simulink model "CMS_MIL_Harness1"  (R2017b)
settings: Solver=FixedStepDiscrete  StartTime=0.0  StopTime=23  FixedStep=0.01  RelTol=1e-3  EnableMultiTasking=on
undefined symbols (not defined in the file): sigbuilder_block
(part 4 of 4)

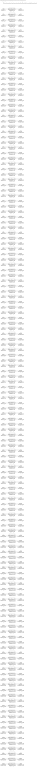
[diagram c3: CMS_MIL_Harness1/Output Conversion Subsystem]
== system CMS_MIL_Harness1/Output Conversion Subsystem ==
  note: This subsystem has been inserted by Simulink to adapt the output of the harnessed component to the interface required by the sink blocks. Modifying the contents of this subsystem may result in compilation and simulation failure.
  Inport_1 : Inport
  Inport_2 : Inport  Port=2
  Inport_3 : Inport  Port=3
  Inport_4 : Inport  Port=4
  Inport_5 : Inport  Port=5
  Inport_6 : Inport  Port=6
  Inport_7 : Inport  Port=7
  Inport_8 : Inport  Port=8
  Inport_9 : Inport  Port=9
  Inport_10 : Inport  Port=10
  Inport_11 : Inport  Port=11
  Inport_12 : Inport  Port=12
  Inport_13 : Inport  Port=13
  Inport_14 : Inport  Port=14
  Inport_15 : Inport  Port=15
  Inport_16 : Inport  Port=16
  Inport_17 : Inport  Port=17
  Inport_18 : Inport  Port=18
  Inport_19 : Inport  Port=19
  Inport_20 : Inport  Port=20
  Inport_21 : Inport  Port=21
  Inport_22 : Inport  Port=22
  Inport_23 : Inport  Port=23
  Inport_24 : Inport  Port=24
  Inport_25 : Inport  Port=25
  Inport_26 : Inport  Port=26
  Inport_27 : Inport  Port=27
  Inport_28 : Inport  Port=28
  Inport_29 : Inport  Port=29
  Inport_30 : Inport  Port=30
  Inport_31 : Inport  Port=31
  Inport_32 : Inport  Port=32
  Inport_33 : Inport  Port=33
  Inport_34 : Inport  Port=34
  Inport_35 : Inport  Port=35
  Inport_36 : Inport  Port=36
  Inport_37 : Inport  Port=37
  Inport_38 : Inport  Port=38
  Inport_39 : Inport  Port=39
  Inport_40 : Inport  Port=40
  Inport_41 : Inport  Port=41
  Inport_42 : Inport  Port=42
  Inport_43 : Inport  Port=43
  Inport_44 : Inport  Port=44
  Inport_45 : Inport  Port=45
  Inport_46 : Inport  Port=46
  Inport_47 : Inport  Port=47
  Inport_48 : Inport  Port=48
  Inport_49 : Inport  Port=49
  Inport_50 : Inport  Port=50
  Inport_51 : Inport  Port=51
  Inport_52 : Inport  Port=52
  Inport_53 : Inport  Port=53
  Inport_54 : Inport  Port=54
  Inport_55 : Inport  Port=55
  Inport_56 : Inport  Port=56
  Inport_57 : Inport  Port=57
  Inport_58 : Inport  Port=58
  Inport_59 : Inport  Port=59
  Inport_60 : Inport  Port=60
  Inport_61 : Inport  Port=61
  Inport_62 : Inport  Port=62
  Inport_63 : Inport  Port=63
  Inport_64 : Inport  Port=64
  Inport_65 : Inport  Port=65
  Inport_66 : Inport  Port=66
  Inport_67 : Inport  Port=67
  Inport_68 : Inport  Port=68
  Inport_69 : Inport  Port=69
  Inport_70 : Inport  Port=70
  Inport_71 : Inport  Port=71
  Inport_72 : Inport  Port=72
  Inport_73 : Inport  Port=73
  Inport_74 : Inport  Port=74
  Inport_75 : Inport  Port=75
  Inport_76 : Inport  Port=76
  Inport_77 : Inport  Port=77
  Inport_78 : Inport  Port=78
  Inport_79 : Inport  Port=79
  Inport_80 : Inport  Port=80
  Inport_81 : Inport  Port=81
  Inport_82 : Inport  Port=82
  Inport_83 : Inport  Port=83
  Inport_84 : Inport  Port=84
  Inport_85 : Inport  Port=85
  Inport_86 : Inport  Port=86
  Inport_87 : Inport  Port=87
  Inport_88 : Inport  Port=88
  Inport_89 : Inport  Port=89
  Inport_90 : Inport  Port=90
  Inport_91 : Inport  Port=91
  Inport_92 : Inport  Port=92
  Inport_93 : Inport  Port=93
  Inport_94 : Inport  Port=94
  Inport_95 : Inport  Port=95
  Inport_96 : Inport  Port=96
  Inport_97 : Inport  Port=97
  Inport_98 : Inport  Port=98
  Inport_99 : Inport  Port=99
  Inport_100 : Inport  Port=100
  Inport_101 : Inport  Port=101
  Inport_102 : Inport  Port=102
  Inport_103 : Inport  Port=103
  Inport_104 : Inport  Port=104
  Inport_105 : Inport  Port=105
  Inport_106 : Inport  Port=106
  Inport_107 : Inport  Port=107
  Inport_108 : Inport  Port=108
  Inport_109 : Inport  Port=109
  Inport_110 : Inport  Port=110
  Inport_111 : Inport  Port=111
  Inport_112 : Inport  Port=112
  Inport_113 : Inport  Port=113
  Inport_114 : Inport  Port=114
  Inport_115 : Inport  Port=115
  Inport_116 : Inport  Port=116
  Inport_117 : Inport  Port=117
  Inport_118 : Inport  Port=118
  Inport_119 : Inport  Port=119
  Inport_120 : Inport  Port=120
  Inport_121 : Inport  Port=121
  Inport_122 : Inport  Port=122
  Inport_123 : Inport  Port=123
  Inport_124 : Inport  Port=124
  Inport_125 : Inport  Port=125
  Inport_126 : Inport  Port=126
  Inport_127 : Inport  Port=127
  Inport_128 : Inport  Port=128
  Inport_129 : Inport  Port=129
  Inport_130 : Inport  Port=130
  Inport_131 : Inport  Port=131
  Inport_132 : Inport  Port=132
  Inport_133 : Inport  Port=133
  Inport_134 : Inport  Port=134
  Inport_135 : Inport  Port=135
  Inport_136 : Inport  Port=136
  Inport_137 : Inport  Port=137
  Inport_138 : Inport  Port=138
  Inport_139 : Inport  Port=139
  Inport_140 : Inport  Port=140
  Inport_141 : Inport  Port=141
  Inport_142 : Inport  Port=142
  Inport_143 : Inport  Port=143
  SigSpec_{1,6,16..17,22,36..38,41..42,46,57..59,66,78,85..87,135..136,138..140,142..143} (26 alike) : SignalSpecification  OutDataTypeStr=uint8  Unit=enum  Dimensions=[1]  SampleTime=0.01
  SigSpec_{2..5,8,10..11,29,34..35,40,49..52,55..56,67..77,79..83,90,92,97} (36 alike) : SignalSpecification  OutDataTypeStr=boolean  Unit=flg  Dimensions=[1]  SampleTime=0.01
  SigSpec_{100..114,119,127..134} (24 alike) : SignalSpecification  OutDataTypeStr=uint8  Unit=numb  Dimensions=[1]  SampleTime=0.01
  SigSpec_{25,28,115..118} (6 alike) : SignalSpecification  OutDataTypeStr=fixdt('ufix16_Sp001')  Unit=V  Dimensions=[1]  SampleTime=0.01
  SigSpec_{12..13,23..24,26..27,88,93..94,120..126} (16 alike) : SignalSpecification  OutDataTypeStr=fixdt('ufix8_Bn40')  Unit=C  Dimensions=[1]  SampleTime=0.01
  SigSpec_137 : SignalSpecification  OutDataTypeStr=boolean  Unit=flag  Dimensions=[1]  SampleTime=0.01
  SigSpec_14 : SignalSpecification  OutDataTypeStr=fixdt('ufix16_Sp1')  Unit=W  Dimensions=[1]  SampleTime=0.01
  SigSpec_141 : SignalSpecification  OutDataTypeStr=boolean  Unit=flag  Dimensions=[1]  SampleTime=0.01
  SigSpec_15 : SignalSpecification  OutDataTypeStr=fixdt('ufix16_Sp1')  Unit=W  Dimensions=[1]  SampleTime=0.01
  SigSpec_18 : SignalSpecification  OutDataTypeStr=fixdt('ufix16_Sp1')  Unit=A  Dimensions=[1]  SampleTime=0.01
  SigSpec_19 : SignalSpecification  OutDataTypeStr=fixdt('ufix16_Sp1_Bn1500')  Unit=A  Dimensions=[1]  SampleTime=0.01
  SigSpec_20 : SignalSpecification  OutDataTypeStr=uint16  Unit=v  Dimensions=[1]  SampleTime=0.01
  SigSpec_21 : SignalSpecification  OutDataTypeStr=uint16  Unit=v  Dimensions=[1]  SampleTime=0.01
  SigSpec_30 : SignalSpecification  OutDataTypeStr=fixdt('ufix16_Sp1')  Unit=KW  Dimensions=[1]  SampleTime=0.01
  SigSpec_{7,31..32,48,98} (5 alike) : SignalSpecification  OutDataTypeStr=fixdt('ufix16_Sp1')  Unit=V  Dimensions=[1]  SampleTime=0.01
  SigSpec_33 : SignalSpecification  OutDataTypeStr=fixdt('ufix16_Sp1_Bn700')  Unit=A  Dimensions=[1]  SampleTime=0.01
  SigSpec_39 : SignalSpecification  OutDataTypeStr=uint8  Unit=%  Dimensions=[1]  SampleTime=0.01
  SigSpec_43 : SignalSpecification  OutDataTypeStr=fixdt('ufix8_B80')  Unit=pct  Dimensions=[1]  SampleTime=0.01
  SigSpec_44 : SignalSpecification  OutDataTypeStr=uint8  Unit=%  Dimensions=[1]  SampleTime=0.01
  SigSpec_45 : SignalSpecification  OutDataTypeStr=uint8  Unit=%  Dimensions=[1]  SampleTime=0.01
  SigSpec_47 : SignalSpecification  OutDataTypeStr=fixdt('ufix16_Bn1023')  Unit=A  Dimensions=[1]  SampleTime=0.01
  SigSpec_53 : SignalSpecification  OutDataTypeStr=fixdt('ufix16_Sp1')  Unit=A  Dimensions=[1]  SampleTime=0.01
  SigSpec_54 : SignalSpecification  OutDataTypeStr=fixdt('ufix16_Sp1_Bn700')  Unit=A  Dimensions=[1]  SampleTime=0.01
  SigSpec_{60..63} (4 alike) : SignalSpecification  OutDataTypeStr=fixdt('ufix16_Sp1')  Unit=kw  Dimensions=[1]  SampleTime=0.01
  SigSpec_64 : SignalSpecification  OutDataTypeStr=uint16  Unit=Kohm  Dimensions=[1]  SampleTime=0.01
  SigSpec_65 : SignalSpecification  OutDataTypeStr=uint16  Unit=min  Dimensions=[1]  SampleTime=0.01
  SigSpec_84 : SignalSpecification  OutDataTypeStr=uint8  Unit=pct  Dimensions=[1]  SampleTime=0.01
  SigSpec_89 : SignalSpecification  OutDataTypeStr=fixdt('ufix16_Sp01')  Unit=Kwh  Dimensions=[1]  SampleTime=0.01
  SigSpec_9 : SignalSpecification  OutDataTypeStr=fixdt('ufix16_Sp1_Bn700')  Unit=A  Dimensions=[1]  SampleTime=0.01
  SigSpec_91 : SignalSpecification  OutDataTypeStr=fixdt('ufix16_Sp1')  Unit=Kwh  Dimensions=[1]  SampleTime=0.01
  SigSpec_95 : SignalSpecification  OutDataTypeStr=fixdt('ufix8_E1')  Unit=V  Dimensions=[1]  SampleTime=0.01
  SigSpec_96 : SignalSpecification  OutDataTypeStr=uint8  Unit=Ah  Dimensions=[1]  SampleTime=0.01
  SigSpec_99 : SignalSpecification  OutDataTypeStr=fixdt('ufix16_Sp1_Bn400')  Unit=A  Dimensions=[1]  SampleTime=0.01
  Outport_1 : Outport
  Outport_2 : Outport  Port=2
  Outport_3 : Outport  Port=3
  Outport_4 : Outport  Port=4
  Outport_5 : Outport  Port=5
  Outport_6 : Outport  Port=6
  Outport_7 : Outport  Port=7
  Outport_8 : Outport  Port=8
  Outport_9 : Outport  Port=9
  Outport_10 : Outport  Port=10
  Outport_11 : Outport  Port=11
  Outport_12 : Outport  Port=12
  Outport_13 : Outport  Port=13
  Outport_14 : Outport  Port=14
  Outport_15 : Outport  Port=15
  Outport_16 : Outport  Port=16
  Outport_17 : Outport  Port=17
  Outport_18 : Outport  Port=18
  Outport_19 : Outport  Port=19
  Outport_20 : Outport  Port=20
  Outport_21 : Outport  Port=21
  Outport_22 : Outport  Port=22
  Outport_23 : Outport  Port=23
  Outport_24 : Outport  Port=24
  Outport_25 : Outport  Port=25
  Outport_26 : Outport  Port=26
  Outport_27 : Outport  Port=27
  Outport_28 : Outport  Port=28
  Outport_29 : Outport  Port=29
  Outport_30 : Outport  Port=30
  Outport_31 : Outport  Port=31
  Outport_32 : Outport  Port=32
  Outport_33 : Outport  Port=33
  Outport_34 : Outport  Port=34
  Outport_35 : Outport  Port=35
  Outport_36 : Outport  Port=36
  Outport_37 : Outport  Port=37
  Outport_38 : Outport  Port=38
  Outport_39 : Outport  Port=39
  Outport_40 : Outport  Port=40
  Outport_41 : Outport  Port=41
  Outport_42 : Outport  Port=42
  Outport_43 : Outport  Port=43
  Outport_44 : Outport  Port=44
  Outport_45 : Outport  Port=45
  Outport_46 : Outport  Port=46
  Outport_47 : Outport  Port=47
  Outport_48 : Outport  Port=48
  Outport_49 : Outport  Port=49
  Outport_50 : Outport  Port=50
  Outport_51 : Outport  Port=51
  Outport_52 : Outport  Port=52
  Outport_53 : Outport  Port=53
  Outport_54 : Outport  Port=54
  Outport_55 : Outport  Port=55
  Outport_56 : Outport  Port=56
  Outport_57 : Outport  Port=57
  Outport_58 : Outport  Port=58
  Outport_59 : Outport  Port=59
  Outport_60 : Outport  Port=60
  Outport_61 : Outport  Port=61
  Outport_62 : Outport  Port=62
  Outport_63 : Outport  Port=63
  Outport_64 : Outport  Port=64
  Outport_65 : Outport  Port=65
  Outport_66 : Outport  Port=66
  Outport_67 : Outport  Port=67
  Outport_68 : Outport  Port=68
  Outport_69 : Outport  Port=69
  Outport_70 : Outport  Port=70
  Outport_71 : Outport  Port=71
  Outport_72 : Outport  Port=72
  Outport_73 : Outport  Port=73
  Outport_74 : Outport  Port=74
  Outport_75 : Outport  Port=75
  Outport_76 : Outport  Port=76
  Outport_77 : Outport  Port=77
  Outport_78 : Outport  Port=78
  Outport_79 : Outport  Port=79
  Outport_80 : Outport  Port=80
  Outport_81 : Outport  Port=81
  Outport_82 : Outport  Port=82
  Outport_83 : Outport  Port=83
  Outport_84 : Outport  Port=84
  Outport_85 : Outport  Port=85
  Outport_86 : Outport  Port=86
  Outport_87 : Outport  Port=87
  Outport_88 : Outport  Port=88
  Outport_89 : Outport  Port=89
  Outport_90 : Outport  Port=90
  Outport_91 : Outport  Port=91
  Outport_92 : Outport  Port=92
  Outport_93 : Outport  Port=93
  Outport_94 : Outport  Port=94
  Outport_95 : Outport  Port=95
  Outport_96 : Outport  Port=96
  Outport_97 : Outport  Port=97
  Outport_98 : Outport  Port=98
  Outport_99 : Outport  Port=99
  Outport_100 : Outport  Port=100
  Outport_101 : Outport  Port=101
  Outport_102 : Outport  Port=102
  Outport_103 : Outport  Port=103
  Outport_104 : Outport  Port=104
  Outport_105 : Outport  Port=105
  Outport_106 : Outport  Port=106
  Outport_107 : Outport  Port=107
  Outport_108 : Outport  Port=108
  Outport_109 : Outport  Port=109
  Outport_110 : Outport  Port=110
  Outport_111 : Outport  Port=111
  Outport_112 : Outport  Port=112
  Outport_113 : Outport  Port=113
  Outport_114 : Outport  Port=114
  Outport_115 : Outport  Port=115
  Outport_116 : Outport  Port=116
  Outport_117 : Outport  Port=117
  Outport_118 : Outport  Port=118
  Outport_119 : Outport  Port=119
  Outport_120 : Outport  Port=120
  Outport_121 : Outport  Port=121
  Outport_122 : Outport  Port=122
  Outport_123 : Outport  Port=123
  Outport_124 : Outport  Port=124
  Outport_125 : Outport  Port=125
  Outport_126 : Outport  Port=126
  Outport_127 : Outport  Port=127
  Outport_128 : Outport  Port=128
  Outport_129 : Outport  Port=129
  Outport_130 : Outport  Port=130
  Outport_131 : Outport  Port=131
  Outport_132 : Outport  Port=132
  Outport_133 : Outport  Port=133
  Outport_134 : Outport  Port=134
  Outport_135 : Outport  Port=135
  Outport_136 : Outport  Port=136
  Outport_137 : Outport  Port=137
  Outport_138 : Outport  Port=138
  Outport_139 : Outport  Port=139
  Outport_140 : Outport  Port=140
  Outport_141 : Outport  Port=141
  Outport_142 : Outport  Port=142
  Outport_143 : Outport  Port=143
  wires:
  Inport_1/1 -> SigSpec_1/1
  SigSpec_1/1 -> Outport_1/1
  Inport_2/1 -> SigSpec_2/1
  SigSpec_2/1 -> Outport_2/1
  Inport_3/1 -> SigSpec_3/1
  SigSpec_3/1 -> Outport_3/1
  Inport_4/1 -> SigSpec_4/1
  SigSpec_4/1 -> Outport_4/1
  Inport_5/1 -> SigSpec_5/1
  SigSpec_5/1 -> Outport_5/1
  Inport_6/1 -> SigSpec_6/1
  SigSpec_6/1 -> Outport_6/1
  Inport_7/1 -> SigSpec_7/1
  SigSpec_7/1 -> Outport_7/1
  Inport_8/1 -> SigSpec_8/1
  SigSpec_8/1 -> Outport_8/1
  Inport_9/1 -> SigSpec_9/1
  SigSpec_9/1 -> Outport_9/1
  Inport_10/1 -> SigSpec_10/1
  SigSpec_10/1 -> Outport_10/1
  Inport_11/1 -> SigSpec_11/1
  SigSpec_11/1 -> Outport_11/1
  Inport_12/1 -> SigSpec_12/1
  SigSpec_12/1 -> Outport_12/1
  Inport_13/1 -> SigSpec_13/1
  SigSpec_13/1 -> Outport_13/1
  Inport_14/1 -> SigSpec_14/1
  SigSpec_14/1 -> Outport_14/1
  Inport_15/1 -> SigSpec_15/1
  SigSpec_15/1 -> Outport_15/1
  Inport_16/1 -> SigSpec_16/1
  SigSpec_16/1 -> Outport_16/1
  Inport_17/1 -> SigSpec_17/1
  SigSpec_17/1 -> Outport_17/1
  Inport_18/1 -> SigSpec_18/1
  SigSpec_18/1 -> Outport_18/1
  Inport_19/1 -> SigSpec_19/1
  SigSpec_19/1 -> Outport_19/1
  Inport_20/1 -> SigSpec_20/1
  SigSpec_20/1 -> Outport_20/1
  Inport_21/1 -> SigSpec_21/1
  SigSpec_21/1 -> Outport_21/1
  Inport_22/1 -> SigSpec_22/1
  SigSpec_22/1 -> Outport_22/1
  Inport_23/1 -> SigSpec_23/1
  SigSpec_23/1 -> Outport_23/1
  Inport_24/1 -> SigSpec_24/1
  SigSpec_24/1 -> Outport_24/1
  Inport_25/1 -> SigSpec_25/1
  SigSpec_25/1 -> Outport_25/1
  Inport_26/1 -> SigSpec_26/1
  SigSpec_26/1 -> Outport_26/1
  Inport_27/1 -> SigSpec_27/1
  SigSpec_27/1 -> Outport_27/1
  Inport_28/1 -> SigSpec_28/1
  SigSpec_28/1 -> Outport_28/1
  Inport_29/1 -> SigSpec_29/1
  SigSpec_29/1 -> Outport_29/1
  Inport_30/1 -> SigSpec_30/1
  SigSpec_30/1 -> Outport_30/1
  Inport_31/1 -> SigSpec_31/1
  SigSpec_31/1 -> Outport_31/1
  Inport_32/1 -> SigSpec_32/1
  SigSpec_32/1 -> Outport_32/1
  Inport_33/1 -> SigSpec_33/1
  SigSpec_33/1 -> Outport_33/1
  Inport_34/1 -> SigSpec_34/1
  SigSpec_34/1 -> Outport_34/1
  Inport_35/1 -> SigSpec_35/1
  SigSpec_35/1 -> Outport_35/1
  Inport_36/1 -> SigSpec_36/1
  SigSpec_36/1 -> Outport_36/1
  Inport_37/1 -> SigSpec_37/1
  SigSpec_37/1 -> Outport_37/1
  Inport_38/1 -> SigSpec_38/1
  SigSpec_38/1 -> Outport_38/1
  Inport_39/1 -> SigSpec_39/1
  SigSpec_39/1 -> Outport_39/1
  Inport_40/1 -> SigSpec_40/1
  SigSpec_40/1 -> Outport_40/1
  Inport_41/1 -> SigSpec_41/1
  SigSpec_41/1 -> Outport_41/1
  Inport_42/1 -> SigSpec_42/1
  SigSpec_42/1 -> Outport_42/1
  Inport_43/1 -> SigSpec_43/1
  SigSpec_43/1 -> Outport_43/1
  Inport_44/1 -> SigSpec_44/1
  SigSpec_44/1 -> Outport_44/1
  Inport_45/1 -> SigSpec_45/1
  SigSpec_45/1 -> Outport_45/1
  Inport_46/1 -> SigSpec_46/1
  SigSpec_46/1 -> Outport_46/1
  Inport_47/1 -> SigSpec_47/1
  SigSpec_47/1 -> Outport_47/1
  Inport_48/1 -> SigSpec_48/1
  SigSpec_48/1 -> Outport_48/1
  Inport_49/1 -> SigSpec_49/1
  SigSpec_49/1 -> Outport_49/1
  Inport_50/1 -> SigSpec_50/1
  SigSpec_50/1 -> Outport_50/1
  Inport_51/1 -> SigSpec_51/1
  SigSpec_51/1 -> Outport_51/1
  Inport_52/1 -> SigSpec_52/1
  SigSpec_52/1 -> Outport_52/1
  Inport_53/1 -> SigSpec_53/1
  SigSpec_53/1 -> Outport_53/1
  Inport_54/1 -> SigSpec_54/1
  SigSpec_54/1 -> Outport_54/1
  Inport_55/1 -> SigSpec_55/1
  SigSpec_55/1 -> Outport_55/1
  Inport_56/1 -> SigSpec_56/1
  SigSpec_56/1 -> Outport_56/1
  Inport_57/1 -> SigSpec_57/1
  SigSpec_57/1 -> Outport_57/1
  Inport_58/1 -> SigSpec_58/1
  SigSpec_58/1 -> Outport_58/1
  Inport_59/1 -> SigSpec_59/1
  SigSpec_59/1 -> Outport_59/1
  Inport_60/1 -> SigSpec_60/1
  SigSpec_60/1 -> Outport_60/1
  Inport_61/1 -> SigSpec_61/1
  SigSpec_61/1 -> Outport_61/1
  Inport_62/1 -> SigSpec_62/1
  SigSpec_62/1 -> Outport_62/1
  Inport_63/1 -> SigSpec_63/1
  SigSpec_63/1 -> Outport_63/1
  Inport_64/1 -> SigSpec_64/1
  SigSpec_64/1 -> Outport_64/1
  Inport_65/1 -> SigSpec_65/1
  SigSpec_65/1 -> Outport_65/1
  Inport_66/1 -> SigSpec_66/1
  SigSpec_66/1 -> Outport_66/1
  Inport_67/1 -> SigSpec_67/1
  SigSpec_67/1 -> Outport_67/1
  Inport_68/1 -> SigSpec_68/1
  SigSpec_68/1 -> Outport_68/1
  Inport_69/1 -> SigSpec_69/1
  SigSpec_69/1 -> Outport_69/1
  Inport_70/1 -> SigSpec_70/1
  SigSpec_70/1 -> Outport_70/1
  Inport_71/1 -> SigSpec_71/1
  SigSpec_71/1 -> Outport_71/1
  Inport_72/1 -> SigSpec_72/1
  SigSpec_72/1 -> Outport_72/1
  Inport_73/1 -> SigSpec_73/1
  SigSpec_73/1 -> Outport_73/1
  Inport_74/1 -> SigSpec_74/1
  SigSpec_74/1 -> Outport_74/1
  Inport_75/1 -> SigSpec_75/1
  SigSpec_75/1 -> Outport_75/1
  Inport_76/1 -> SigSpec_76/1
  SigSpec_76/1 -> Outport_76/1
  Inport_77/1 -> SigSpec_77/1
  SigSpec_77/1 -> Outport_77/1
  Inport_78/1 -> SigSpec_78/1
  SigSpec_78/1 -> Outport_78/1
  Inport_79/1 -> SigSpec_79/1
  SigSpec_79/1 -> Outport_79/1
  Inport_80/1 -> SigSpec_80/1
  SigSpec_80/1 -> Outport_80/1
  Inport_81/1 -> SigSpec_81/1
  SigSpec_81/1 -> Outport_81/1
  Inport_82/1 -> SigSpec_82/1
  SigSpec_82/1 -> Outport_82/1
  Inport_83/1 -> SigSpec_83/1
  SigSpec_83/1 -> Outport_83/1
  Inport_84/1 -> SigSpec_84/1
  SigSpec_84/1 -> Outport_84/1
  Inport_85/1 -> SigSpec_85/1
  SigSpec_85/1 -> Outport_85/1
  Inport_86/1 -> SigSpec_86/1
  SigSpec_86/1 -> Outport_86/1
  Inport_87/1 -> SigSpec_87/1
  SigSpec_87/1 -> Outport_87/1
  Inport_88/1 -> SigSpec_88/1
  SigSpec_88/1 -> Outport_88/1
  Inport_89/1 -> SigSpec_89/1
  SigSpec_89/1 -> Outport_89/1
  Inport_90/1 -> SigSpec_90/1
  SigSpec_90/1 -> Outport_90/1
  Inport_91/1 -> SigSpec_91/1
  SigSpec_91/1 -> Outport_91/1
  Inport_92/1 -> SigSpec_92/1
  SigSpec_92/1 -> Outport_92/1
  Inport_93/1 -> SigSpec_93/1
  SigSpec_93/1 -> Outport_93/1
  Inport_94/1 -> SigSpec_94/1
  SigSpec_94/1 -> Outport_94/1
  Inport_95/1 -> SigSpec_95/1
  SigSpec_95/1 -> Outport_95/1
  Inport_96/1 -> SigSpec_96/1
  SigSpec_96/1 -> Outport_96/1
  Inport_97/1 -> SigSpec_97/1
  SigSpec_97/1 -> Outport_97/1
  Inport_98/1 -> SigSpec_98/1
  SigSpec_98/1 -> Outport_98/1
  Inport_99/1 -> SigSpec_99/1
  SigSpec_99/1 -> Outport_99/1
  Inport_100/1 -> SigSpec_100/1
  SigSpec_100/1 -> Outport_100/1
  Inport_101/1 -> SigSpec_101/1
  SigSpec_101/1 -> Outport_101/1
  Inport_102/1 -> SigSpec_102/1
  SigSpec_102/1 -> Outport_102/1
  Inport_103/1 -> SigSpec_103/1
  SigSpec_103/1 -> Outport_103/1
  Inport_104/1 -> SigSpec_104/1
  SigSpec_104/1 -> Outport_104/1
  Inport_105/1 -> SigSpec_105/1
  SigSpec_105/1 -> Outport_105/1
  Inport_106/1 -> SigSpec_106/1
  SigSpec_106/1 -> Outport_106/1
  Inport_107/1 -> SigSpec_107/1
  SigSpec_107/1 -> Outport_107/1
  Inport_108/1 -> SigSpec_108/1
  SigSpec_108/1 -> Outport_108/1
  Inport_109/1 -> SigSpec_109/1
  SigSpec_109/1 -> Outport_109/1
  Inport_110/1 -> SigSpec_110/1
  SigSpec_110/1 -> Outport_110/1
  Inport_111/1 -> SigSpec_111/1
  SigSpec_111/1 -> Outport_111/1
  Inport_112/1 -> SigSpec_112/1
  SigSpec_112/1 -> Outport_112/1
  Inport_113/1 -> SigSpec_113/1
  SigSpec_113/1 -> Outport_113/1
  Inport_114/1 -> SigSpec_114/1
  SigSpec_114/1 -> Outport_114/1
  Inport_115/1 -> SigSpec_115/1
  SigSpec_115/1 -> Outport_115/1
  Inport_116/1 -> SigSpec_116/1
  SigSpec_116/1 -> Outport_116/1
  Inport_117/1 -> SigSpec_117/1
  SigSpec_117/1 -> Outport_117/1
  Inport_118/1 -> SigSpec_118/1
  SigSpec_118/1 -> Outport_118/1
  Inport_119/1 -> SigSpec_119/1
  SigSpec_119/1 -> Outport_119/1
  Inport_120/1 -> SigSpec_120/1
  SigSpec_120/1 -> Outport_120/1
  Inport_121/1 -> SigSpec_121/1
  SigSpec_121/1 -> Outport_121/1
  Inport_122/1 -> SigSpec_122/1
  SigSpec_122/1 -> Outport_122/1
  Inport_123/1 -> SigSpec_123/1
  SigSpec_123/1 -> Outport_123/1
  Inport_124/1 -> SigSpec_124/1
  SigSpec_124/1 -> Outport_124/1
  Inport_125/1 -> SigSpec_125/1
  SigSpec_125/1 -> Outport_125/1
  Inport_126/1 -> SigSpec_126/1
  SigSpec_126/1 -> Outport_126/1
  Inport_127/1 -> SigSpec_127/1
  SigSpec_127/1 -> Outport_127/1
  Inport_128/1 -> SigSpec_128/1
  SigSpec_128/1 -> Outport_128/1
  Inport_129/1 -> SigSpec_129/1
  SigSpec_129/1 -> Outport_129/1
  Inport_130/1 -> SigSpec_130/1
  SigSpec_130/1 -> Outport_130/1
  Inport_131/1 -> SigSpec_131/1
  SigSpec_131/1 -> Outport_131/1
  Inport_132/1 -> SigSpec_132/1
  SigSpec_132/1 -> Outport_132/1
  Inport_133/1 -> SigSpec_133/1
  SigSpec_133/1 -> Outport_133/1
  Inport_134/1 -> SigSpec_134/1
  SigSpec_134/1 -> Outport_134/1
  Inport_135/1 -> SigSpec_135/1
  SigSpec_135/1 -> Outport_135/1
  Inport_136/1 -> SigSpec_136/1
  SigSpec_136/1 -> Outport_136/1
  Inport_137/1 -> SigSpec_137/1
  SigSpec_137/1 -> Outport_137/1
  Inport_138/1 -> SigSpec_138/1
  SigSpec_138/1 -> Outport_138/1
  Inport_139/1 -> SigSpec_139/1
  SigSpec_139/1 -> Outport_139/1
  Inport_140/1 -> SigSpec_140/1
  SigSpec_140/1 -> Outport_140/1
  Inport_141/1 -> SigSpec_141/1
  SigSpec_141/1 -> Outport_141/1
  Inport_142/1 -> SigSpec_142/1
  SigSpec_142/1 -> Outport_142/1
  Inport_143/1 -> SigSpec_143/1
  SigSpec_143/1 -> Outport_143/1
